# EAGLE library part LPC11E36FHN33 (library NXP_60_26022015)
32-bit ARM Cortex-M0 microcontroller; up to 128 kB flash; up to 12 kB SRAM and 4 kB EEPROM; USART The LPC11E3x are a ARM Cortex-M0 based, low-cost 32-bit MCU family, designed for 8/16-bit microcontroller applications, offering performance, low power, simple instruction set and memory addressing together with reduced code size compared to existing 8/16-bit architectures. The LPC11E3x operate at CPU frequencies of up to 50 MHz. The peripheral complement of the LPC11E3x includes up to 128 kB of flash memory, up to 12 kB of SRAM data memory and 4 kB EEPROM, one Fast-mode Plus I 2 C-bus interface, one RS-485/EIA-485 USART with support for synchronous mode and smart card interface, two SSP interfaces, four general purpose counter/timers, a 10-bit ADC, and up to 54 general purpose I/O pins. AAL Eindhoven MK
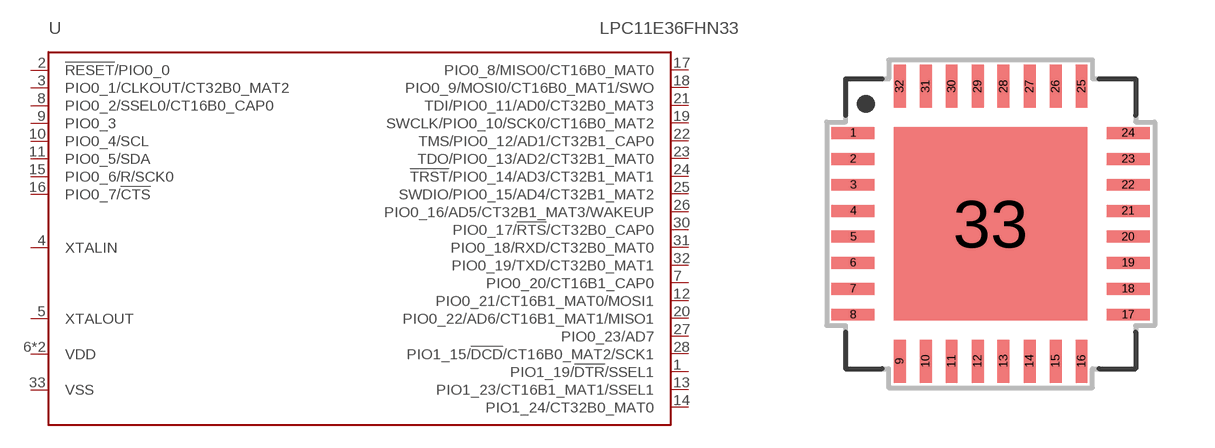
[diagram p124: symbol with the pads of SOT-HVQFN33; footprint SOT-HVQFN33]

Designator prefix U

## LPC11E36FHN33  [SOT-HVQFN33]
1  PIO1_19/!DTR!/SSEL1
2  !RESET!/PIO0_0
3  PIO0_1/CLKOUT/CT32B0_MAT2
4  XTALIN  in
5  XTALOUT  out
6  VDD  pwr
7  PIO0_20/CT16B1_CAP0
8  PIO0_2/SSEL0/CT16B0_CAP0
9  PIO0_3
10  PIO0_4/SCL
11  PIO0_5/SDA
12  PIO0_21/CT16B1_MAT0/MOSI1
13  PIO1_23/CT16B1_MAT1/SSEL1
14  PIO1_24/CT32B0_MAT0
15  PIO0_6/R/SCK0
16  PIO0_7/!CTS!
17  PIO0_8/MISO0/CT16B0_MAT0
18  PIO0_9/MOSI0/CT16B0_MAT1/SWO
19  SWCLK/PIO0_10/SCK0/CT16B0_MAT2
20  PIO0_22/AD6/CT16B1_MAT1/MISO1
21  TDI/PIO0_11/AD0/CT32B0_MAT3
22  TMS/PIO0_12/AD1/CT32B1_CAP0
23  TDO/PIO0_13/AD2/CT32B1_MAT0
24  !TRST!/PIO0_14/AD3/CT32B1_MAT1
25  SWDIO/PIO0_15/AD4/CT32B1_MAT2
26  PIO0_16/AD5/CT32B1_MAT3/WAKEUP
27  PIO0_23/AD7
28  PIO1_15/!DCD!/CT16B0_MAT2/SCK1
29  VDD  pwr
30  PIO0_17/!RTS!/CT32B0_CAP0
31  PIO0_18/RXD/CT32B0_MAT0
32  PIO0_19/TXD/CT32B0_MAT1
33  VSS  pwr

## Footprint SOT-HVQFN33 (pad centres in mm)
SOTxxx HVQFN33: plastic thermal enhanced very thin quad flat package; no leads; 33 terminals; body 7 x 7 x 0.85 mm JEDEC: --- IEC: --- Package according LPC111x datasheet
smd 1.075 x 0.3: 1 -3.438,2.275; 2 -3.438,1.625; 3 -3.438,0.975; 4 -3.438,0.325; 5 -3.438,-0.325; 6 -3.438,-0.975; 7 -3.438,-1.625; 8 -3.438,-2.275; 17 3.438,-2.275; 18 3.438,-1.625; 19 3.438,-0.975; 20 3.438,-0.325; 21 3.438,0.325; 22 3.438,0.975; 23 3.438,1.625; 24 3.438,2.275
smd 0.3 x 1.075: 9 -2.275,-3.438; 10 -1.625,-3.438; 11 -0.975,-3.438; 12 -0.325,-3.438; 13 0.325,-3.438; 14 0.975,-3.438; 15 1.625,-3.438; 16 2.275,-3.438; 25 2.275,3.438; 26 1.625,3.438; 27 0.975,3.438; 28 0.325,3.438; 29 -0.325,3.438; 30 -0.975,3.438; 31 -1.625,3.438; 32 -2.275,3.438
smd 4.85 x 4.85: 33 0,0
